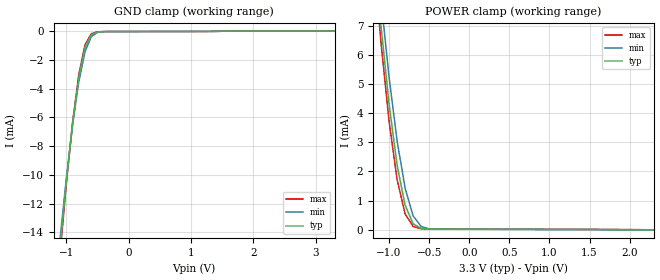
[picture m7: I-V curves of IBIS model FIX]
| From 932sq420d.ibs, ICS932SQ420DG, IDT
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|   Model FIX
[Model]   FIX
Model_type   Input
Polarity   Non-Inverting
Vinl =   0.80V
Vinh =   2.00V
C_comp   3.40pF   2.85pF   3.95pF
[Temperature Range]   27.00   70.00   0.000
[Voltage Range]   3.30V   3.00V   3.70V
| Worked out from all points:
|   GND clamp passes 1 mA (typ) near -0.69 V on its own axis
|   POWER clamp passes 1 mA (typ) near -0.81 V on its own axis
[GND_clamp]
| voltage   I(typ)   I(min)   I(max)
-3.3V     -140mA     -130mA     -150mA
-1.1V     -15.06mA   -14.43mA   -15.54mA
-1V       -10.47mA   -10.26mA   -10.64mA
-900mV    -6.45mA    -6.56mA    -6.37mA
-800mV    -3.23mA    -3.53mA    -3.01mA
-700mV    -1.13mA    -1.42mA    -940uA
-600mV    -240uA     -380uA     -170uA
-500mV    -45.93uA   -76.06uA   -35.4uA
-400mV    -20.06uA   -23.55uA   -20.53uA
3.3V      15.02uA    15.15uA    15.02uA
[POWER_clamp]
| voltage   I(typ)   I(min)   I(max)
-3.3V     150mA      140mA      150mA
-1.2V     10.13mA    10.93mA    9.65mA
-1.1V     6.98mA     7.88mA     6.4mA
-1V       4.31mA     5.24mA     3.72mA
-900mV    2.22mA     3.05mA     1.72mA
-800mV    840uA      1.43mA     540uA
-700mV    200uA      470uA      110uA
-600mV    42.64uA    110uA      28.63uA
-500mV    19.91uA    29.2uA     20uA
2.3V      -10.4uA    -10.91uA   -6.15uA
